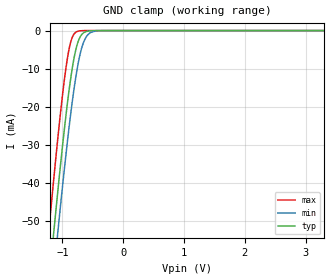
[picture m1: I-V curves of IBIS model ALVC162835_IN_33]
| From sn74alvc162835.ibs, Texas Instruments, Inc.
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[Model]   ALVC162835_IN_33
Model_type  Input
Vinl=0.8
Vinh=2.0
| variable   typ   min   max
C_comp   10.88pF   10.57pF   11.06pF
[Temperature Range]   40   100   -40
| Ambient temperature   25   85   -40
[Voltage range]   3.3   3   3.6
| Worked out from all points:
|   GND clamp passes 1 mA (typ) near -0.68 V on its own axis
[GND Clamp]
| ALVC162835_IN_33
|   Voltage   I(typ)   I(min)   I(max)
-3.3V     -451.4mA   -460.2mA   -440.6mA
-1.225V   -66.77mA   -77.63mA   -52.81mA
-1.14V    -52.55mA   -63.42mA   -38.55mA
-1.07V    -41.27mA   -52.08mA   -27.39mA
-975mV    -26.91mA   -37.4mA    -13.81mA
-905mV    -17.45mA   -27.36mA   -6.068mA
-845mV    -10.58mA   -19.54mA   -2.069mA
-765mV    -4.1mA     -10.78mA   -298.6uA
-700mV    -1.444mA   -5.604mA   -52.39uA
-640mV    -472.1uA   -2.617mA   -10.24uA
-470mV    -15.62uA   -178.3uA   -98.78nA
3.3V      1.114nA    59.61nA    6.193pA
